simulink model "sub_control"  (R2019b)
settings: Solver=VariableStepAuto  StartTime=0.0  StopTime=10.0  RelTol=1e-3
libraries: simulink x2

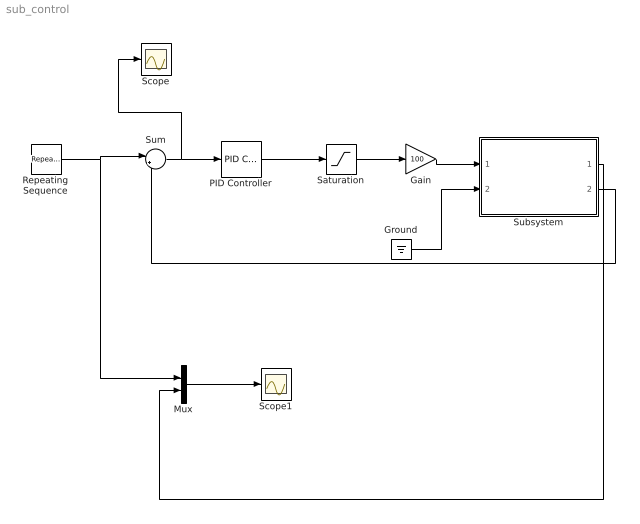
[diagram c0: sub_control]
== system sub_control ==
  Gain : Gain  Gain=100
  Ground : Ground
  Mux : Mux  Inputs=2
  PID Controller : simulink/Continuous/PID Controller  Controller=PID  Form=Parallel  TimeDomain=Continuous-time  SampleTime=-1  IntegratorMethod=Forward Euler  FilterMethod=Forward Euler  ControllerParametersSource=internal  P=1  I=0  D=0  UseFilter=on  N=100  TunerSelectOption=Transfer Function Based (PID Tuner App)  InitialConditionSource=internal  InitialConditionForIntegrator=0  InitialConditionForFilter=0  DifferentiatorICPrevScaledInput=0  ExternalReset=none  TrackingMode=off  Kt=1  LimitOutput=off  UpperSaturationLimit=inf  LowerSaturationLimit=-inf  LinearizeAsGain=on  AntiWindupMode=none  Kb=1  POutMin=[]  POutMax=[]  IOutMin=[]  IOutMax=[]  DOutMin=[]  DOutMax=[]  NOutMin=[]  NOutMax=[]  SumOutMin=[]  SumOutMax=[]  SaturationOutMin=[]  SaturationOutMax=[]  PParamMin=[]  PParamMax=[]  IParamMin=[]  IParamMax=[]  DParamMin=[]  DParamMax=[]  NParamMin=[]  NParamMax=[]  KbParamMin=[]  KbParamMax=[]  KtParamMin=[]  KtParamMax=[]  KbOutMin=[]  KbOutMax=[]  KtOutMin=[]  KtOutMax=[]  IntegratorOutMin=[]  IntegratorOutMax=[]  FilterOutMin=[]  FilterOutMax=[]  SumI1OutMin=[]  SumI1OutMax=[]  SumI2OutMin=[]  SumI2OutMax=[]  SumI3OutMin=[]  SumI3OutMax=[]  SumI4OutMin=[]  SumI4OutMax=[]  SumDOutMin=[]  SumDOutMax=[]  DifferentiatorOutMin=[]  DifferentiatorOutMax=[]  FilterDiffOutCoefMin=[]  FilterDiffOutCoefMax=[]  ReciprocalOutMin=[]  ReciprocalOutMax=[]  SumDenOutMin=[]  SumDenOutMax=[]  SumNumOutMin=[]  SumNumOutMax=[]  DivideOutMin=[]  DivideOutMax=[]  IntegratorContinuousStateAttributes=''  IntegratorStateMustResolveToSignalObject=off  IntegratorRTWStateStorageClass=Auto  FilterContinuousStateAttributes=''  FilterStateMustResolveToSignalObject=off  FilterRTWStateStorageClass=Auto  ParallelPVariant=InternalParameters  IdealPVariant=Disabled  IVariant=InternalParameters  DVariant=InternalParameters  IntegratorVariant=Continuous  SatVariant=Disabled  AWVariant=Passthrough  PCopyVariant=Disabled  TRVariant=Disabled  FdbkBlocksVariant=Forward  IdealPFdbkVariant=Disabled  SatFdbkVariant=Disabled  DerivativeFilterVariant=ContFilter  NVariant=InternalParameters  NCopyVariant=Disabled  FilterICVariant=InternalICsFilter  IntegratorICVariant=InternalICs  ExternalResetVariant=Disabled  TRSumVariant=Passthrough  SumFdbkVariant=Disabled  SumVariant=Sum_PID
  Repeating Sequence : simulink/Sources/Repeating Sequence  rep_seq_t=[0 3 5 8 10]  rep_seq_y=[0 10 5 5 0]
  Saturation : Saturate  UpperLimit=1  LowerLimit=-1
  Scope : Scope
  Scope1 : Scope
  Subsystem : Subsystem
  Sum : Sum  Inputs=|+-
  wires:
  Repeating Sequence/1 -> Mux/1, Sum/1
  Sum/1 -> Scope/1, PID Controller/1
  PID Controller/1 -> Saturation/1
  Saturation/1 -> Gain/1
  Gain/1 -> Subsystem/1(f1)
  Ground/1 -> Subsystem/2(f2)
  Subsystem/2(v2) -> Sum/2
  Subsystem/1(v1) -> Mux/2
  Mux/1 -> Scope1/1

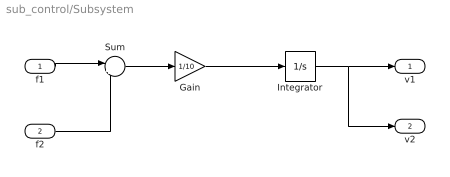
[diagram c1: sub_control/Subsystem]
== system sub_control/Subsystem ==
  f1 : Inport
  f2 : Inport  Port=2
  Gain : Gain  Gain=1/10
  Integrator : Integrator
  Sum : Sum  Inputs=|++
  v1 : Outport
  v2 : Outport  Port=2
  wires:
  f1/1 -> Sum/1
  f2/1 -> Sum/2
  Sum/1 -> Gain/1
  Gain/1 -> Integrator/1
  Integrator/1 -> v2/1, v1/1
